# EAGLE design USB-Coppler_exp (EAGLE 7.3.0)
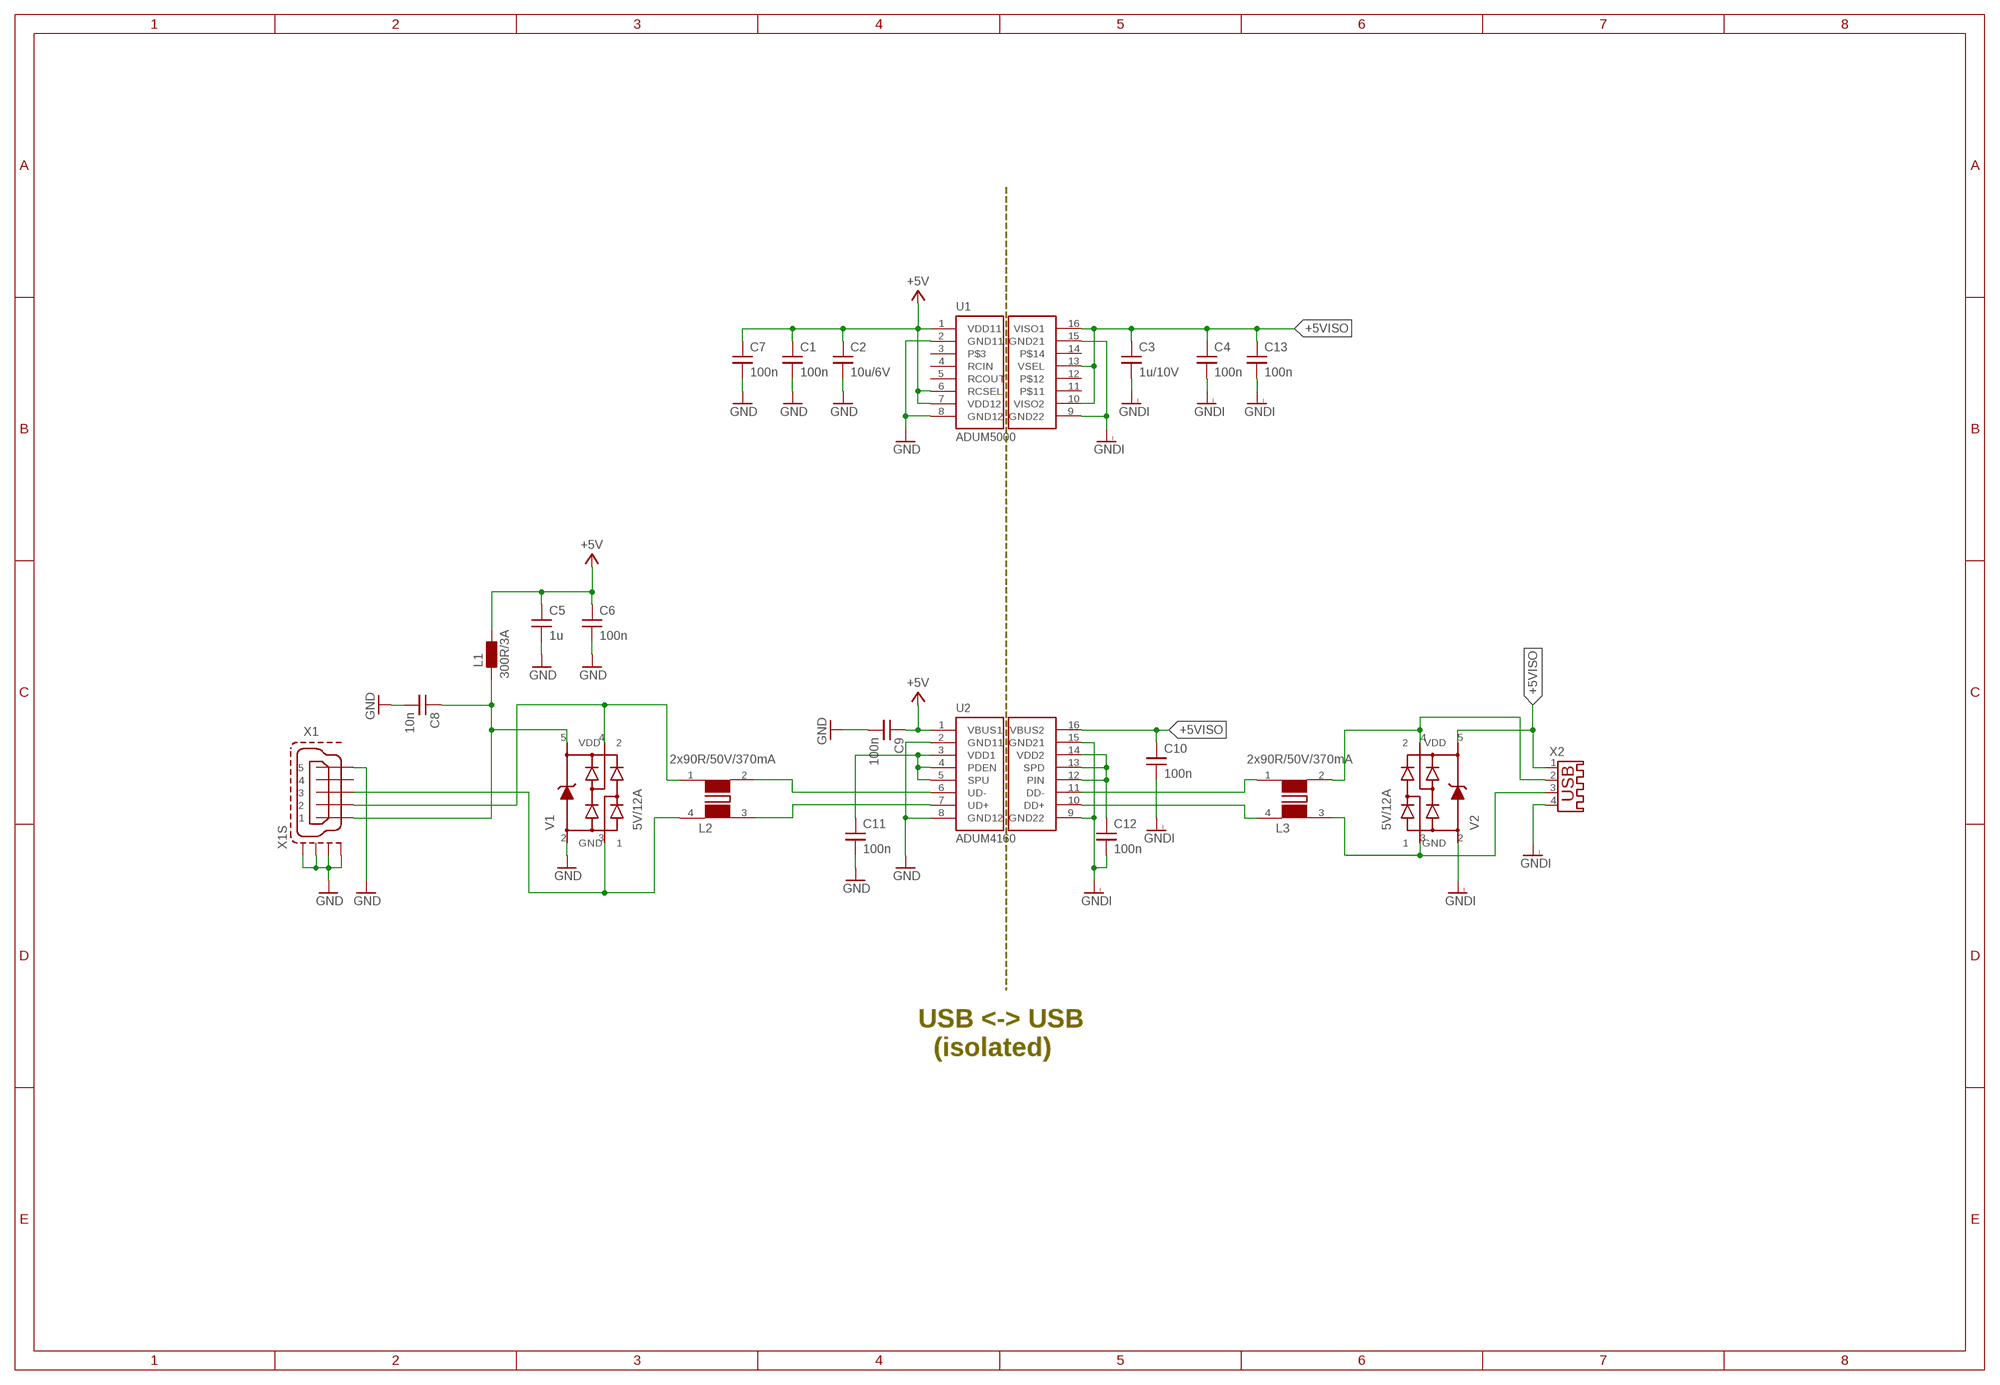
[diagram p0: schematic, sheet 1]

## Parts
C1  100n  C-EUC0603K  [C0603K]
C2  10u/6V  C-EUC0603K  [C0603K]
C3  1u/10V  C-EUC0603K  [C0603K]
C4  100n  C-EUC0603K  [C0603K]
C5  1u  C-EUC0603K  [C0603K]
C6  100n  C-EUC0603K  [C0603K]
C7  100n  C-EUC0603K  [C0603K]
C8  10n  C-EUC0603K  [C0603K]
C9  100n  C-EUC0603K  [C0603K]
C10  100n  C-EUC0603K  [C0603K]
C11  100n  C-EUC0603K  [C0603K]
C12  100n  C-EUC0603K  [C0603K]
C13  100n  C-EUC0603K  [C0603K]
L1  300R/3A  FERRIT-300R_3A  [0805]
L2  2x90R/50V/370mA  FILTER-C-WE-CNSW-1206_90R  [WE-CNSW_1206]
L3  2x90R/50V/370mA  FILTER-C-WE-CNSW-1206_90R  [WE-CNSW_1206]
U1  ADUM5000  [SOIC-16]
U2  ADUM4160  [SOIC-16]
V1  5V/12A  TVS_DIODE_WE-TVS_824011  [SOT23-5]
V2  5V/12A  TVS_DIODE_WE-TVS_824011  [SOT23-5]
X1  XB_MINIUSB_2486-01  [LUMBERG_2486_01]
X2  USB-A003  [USB-A003]

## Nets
+5V: C1.1 C2.1 C5.1 C6.1 C7.1 C9.1 L1.2 U1.1(VDD11) U1.6(RCSEL) U1.7(VDD12) U2.1(VBUS1)
+5VISO: C3.1 C4.1 C10.1 C13.1 U1.10(VISO2) U1.13(VSEL) U1.16(VISO1) U2.16(VBUS2) V2.5(VDD) X2.1
GND: C1.2 C2.2 C5.2 C6.2 C7.2 C8.2 C9.2 C11.2 U1.2(GND11) U1.8(GND12) U2.2(GND11) U2.8(GND12) V1.2(GND) X1.5 X1.M1(S1) X1.M2(S2) X1.M3(S3) X1.M4(S4)
GNDI: C3.2 C4.2 C10.2 C12.2 C13.2 U1.9(GND22) U1.15(GND21) U2.9(GND22) U2.15(GND21) V2.2(GND) X2.4
N$1: C11.1 U2.3(VDD1) U2.4(PDEN) U2.5(SPU)
N$2: L2.2 U2.6(UD-)
N$3: L2.3 U2.7(UD+)
N$5: C12.1 U2.12(PIN) U2.13(SPD) U2.14(VDD2)
N$6: L3.1 U2.11(DD-)
N$7: L3.4 U2.10(DD+)
N$8: L3.3 V2.3 X2.3
N$9: L3.2 V2.4 X2.2
N$531: L2.1 V1.4 X1.2
N$532: L2.4 V1.3 X1.3
N$533: C8.1 L1.1 V1.5(VDD) X1.1
Unconnected: U1.3 U1.4(RCIN) U1.5(RCOUT) U1.11 U1.12 U1.14 X1.4

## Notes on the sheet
- USB <-> USB
    (isolated)

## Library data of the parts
C1-C13 = LV_LG:C-EU: CAPACITOR, European symbol
L1 = 003-Schutzelemente:FERRIT; ARTIKELNR: 50107688; BEZEICHNUNG: Ferrit-C 300R@100MHz 3A 50mR; BEZEICHNUNG2: 742792031; HERSTELLER: WÜRTH
L2 L3 = 008-Filter:FILTER-C: SMD Common Mode Noise Suppressor WE_CNSW - Common mode data line filter - Wire wound -- USB 2.0 -- IEEE 1394 -- Power supply systems -- Signal interfaces; BEZEICHNUNG: Filter-C Datenleitungs-Filter (USB); BEZEICHNUNG2: 744232090; HERSTELLER: Würth
U1 = LV_LG:ADUM5000: FEATURES isoPower integrated, isolated dc-to-dc converter Regulated 3.3 V or 5 V output Up to 500 mW output power 16-lead SOIC package with 7.6 mm creepage High temperature operation: 105°C maximum Thermal overload protection
U2 = LV_LG:ADUM4160: FEATURES USB 2.0 compatible Low and full speed data rate: 1.5 Mbps and 12 Mbps Bidirectional communication 4.5 V to 5.5 V VBUSoperation 7 mA maximum upstream supply current @ 1.5 Mbps 8 mA maximum upstream supply current @ 12 Mbps 2.3 mA maximum upstream idle current Upstream short-circuit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
V1 V2 = 004-Dioden:TVS_DIODE_WE-TVS; ARTIKELNR: 50113145; BEZEICHNUNG: Diode-C WE-TVS Array; BEZEICHNUNG2: 824011 ESD-Protection; HERSTELLER: WUERTH
X1 = 009-Stecker:XB_MINIUSB_2486-01: MINI USB Connector Source: http://www.hirose.co.jp/cataloge_hp/e24000019.pdf; ARTIKELNR: n.v.; BEZEICHNUNG: Buchse Mini USB-B; BEZEICHNUNG2: 2486-01 (Bürklin 72F2280); HERSTELLER: Lumberg
X2 = con-yamaichi:USB-A003: USB connector; OC_FARNELL: unknown; OC_NEWARK: unknown

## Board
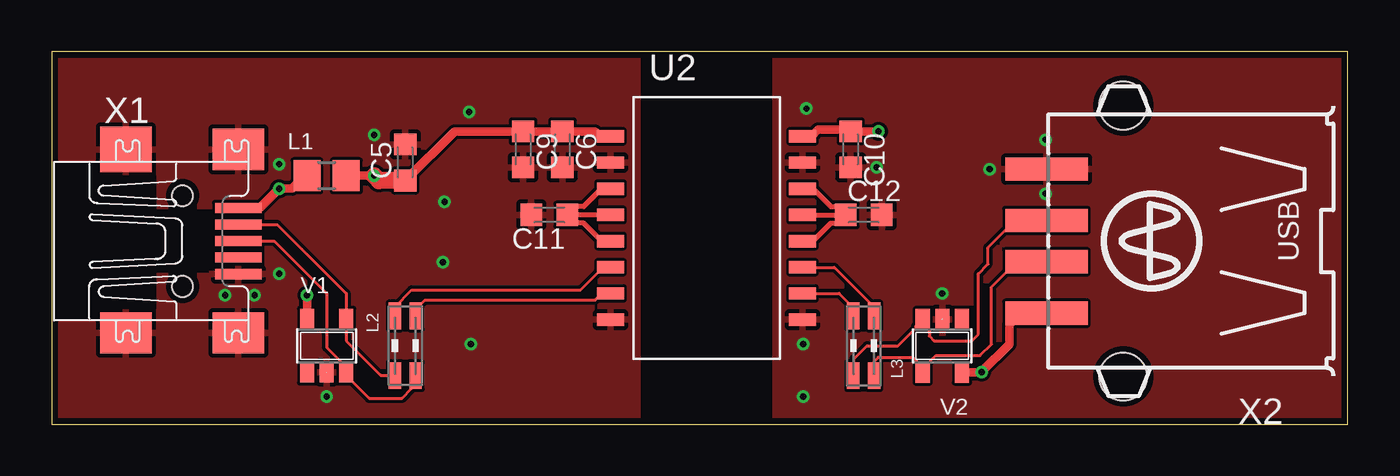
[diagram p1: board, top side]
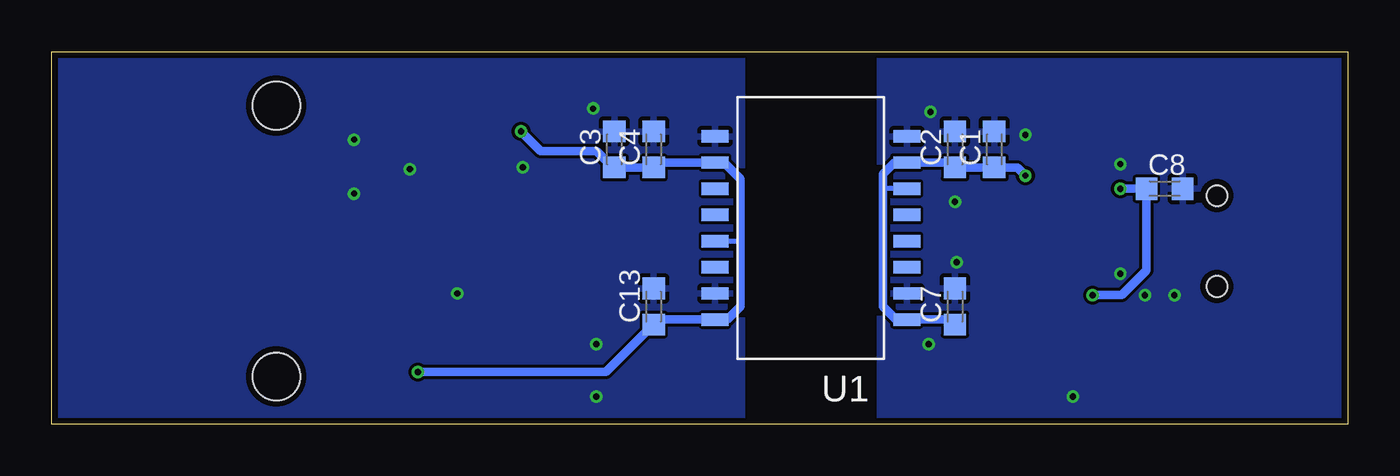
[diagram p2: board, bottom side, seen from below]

Size 62.84 x 18.09 mm. Coordinates in mm from the lower left corner, seen from the top.
Outline: 0,0 62.84,0 62.84,18.09 0,18.09 0,0
Copper layers (1*16): Top 0.035mm / dielectric 1.5mm / Bottom 0.035mm
Design rules "PCB-POOL Standard": minimum track width 0.15mm, minimum drill 0.3mm, track to track 0.15mm, track to pad 0.15mm, pad to pad 0.15mm, via to via 0.15mm, smd to smd 0.15mm, copper to edge 0.3mm, drill to drill 0.2mm, minimum pad ring 0.2mm, minimum via ring 0.15mm, stop-mask expansion 0.075mm, vias tented up to drill 0mil, thermal gap 0.2mm
tRestrict: area 28.6,0 to 34.9,18.4
bRestrict: area 22.9,0 to 29.2,18.4

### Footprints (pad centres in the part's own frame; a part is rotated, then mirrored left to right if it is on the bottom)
C0603K = smd 1.05 x 1.08: 1 -0.875,0; 2 0.875,0
0805 = smd 1.3 x 1.5: 1 -0.95,0; 2 0.95,0
WE-CNSW_1206 = smd 0.6 x 1.3: 1 -0.5,-1.45; 2 -0.5,1.45; 3 0.5,1.45; 4 0.5,-1.45
SOIC-16 = smd 0.6 x 1.3: 1 -4.445,-4.65; 2 -3.175,-4.65; 3 -1.905,-4.65; 4 -0.635,-4.65; 5 0.635,-4.65; 6 1.905,-4.65; 7 3.175,-4.65; 8 4.445,-4.65; 9 4.445,4.65; 10 3.175,4.65; 11 1.905,4.65; 12 0.635,4.65; 13 -0.635,4.65; 14 -1.905,4.65; 15 -3.175,4.65; 16 -4.445,4.65
SOT23-5 = smd 0.69 x 0.99: 1 -0.95,-1.29; 2 0,-1.29; 3 0.95,-1.29; 4 0.95,1.3; 5 -0.95,1.3
LUMBERG_2486_01 = smd 2.25 x 0.5: 1 2.7,1.6; 2 2.7,0.8; 3 2.7,0; 4 2.7,-0.8; 5 2.7,-1.6 | smd 2.5 x 2: M1 -2.75,-4.45; M3 2.7,4.45; M4 2.7,-4.45 | smd 2.5 x 2.2: M2 -2.75,4.45 | hole 1: 0,-2.2; 0,2.2
USB-A003 = smd 1.12 x 4: 1 -3.5,14; 2 -1,14; 3 1,14; 4 3.5,14 | hole 2.3: -6.57,10.28; 6.57,10.28

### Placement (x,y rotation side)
C1  17.14,13.34 90 bottom
C2  19.05,13.34 90 bottom
C3  35.56,13.34 90 bottom
C4  33.66,13.34 90 bottom
C5  17.14,12.7 90 top
C6  24.77,13.34 270 top
C7  19.05,5.71 90 bottom
C8  8.89,11.43 0 bottom
C9  22.86,13.34 270 top
C10  38.73,13.34 270 top
C11  24.13,10.16 180 top
C12  39.37,10.16 0 top
C13  33.66,5.71 90 bottom
L1  13.34,12.06 0 top
L2  17.14,3.81 0 top
L3  39.37,3.81 180 top
U1  26.04,9.53 90 bottom
U2  31.75,9.53 270 top
V1  13.34,3.81 0 top
V2  43.18,3.81 180 top
X1  6.35,8.89 0 top
X2  62.23,8.89 90 top

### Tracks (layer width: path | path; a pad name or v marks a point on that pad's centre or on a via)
+5V  (via drill 0.3)
  Top 0.406: L1.2 v15.64,12.06 | U2.1 26.59,13.97 26.35,14.21 C6.1 C9.1 19.53,14.21 C5.1
  Top 0.813: C5.1 15.88,11.82 v15.64,12.06
  Bottom 0.254: U1.6 22.54,11.43
  Bottom 0.406: v15.64,12.06 16.03,12.46 C1.1 C2.1 19.29,12.7 U1.7 21.99,12.7 22.54,12.14 22.54,11.43 22.54,5.71 21.91,5.08 U1.1 19.29,5.08 C7.1
+5VISO  (via drill 0.3)
  Top 0.406: v40.08,14.21 C10.1 38.66,14.29 37.15,14.29 36.83,13.97 U2.16 | V2.5 45.05,2.51 v45.09,2.54 46.43,3.89 46.43,4.84 46.98,5.39 X2.1
  Bottom 0.254: U1.13 29.45,8.89
  Bottom 0.406: v40.08,14.21 39.13,13.26 36.43,13.26 35.64,12.46 C3.1 C4.1 33.41,12.7 U1.10 30.24,12.7 29.45,11.91 29.45,8.89 29.45,5.71 30.08,5.08 U1.16 33.41,5.08 C13.1 35.96,2.54 v45.09,2.54
GND  (via drill 0.3)
  other vias: 15.64,14.05 11.03,12.62 11.03,7.3 9.84,6.27 8.41,6.27 18.97,7.86 20.32,3.89 20.24,15.16 19.05,10.79 13.34,1.35
  pour Top: 0,0 0,18.41 29.21,18.41 29.21,0
  pour Bottom: 0,0 0,18.41 23.5,18.41 23.5,0
GNDI  (via drill 0.3)
  other vias: 43.18,6.35 45.48,12.38 48.18,13.81 48.18,11.19 36.59,15.32 40.01,12.46 36.43,3.89 36.43,1.35
  pour Bottom: 28.57,0 28.57,18.41 62.87,18.41 62.87,0
  pour Top: 34.29,0 34.29,18.41 62.87,18.41 62.87,0
N$1
  Top 0.254: U2.5 26.67,8.89 25.8,9.76 25.4,9.76 C11.1 | U2.4 C11.1 | U2.3 26.67,11.43 25.8,10.56 25.32,10.56 C11.1
N$2
  Top 0.15: L2.2 16.64,5.69 17.46,6.51 25.64,6.51 26.51,7.38 26.51,7.46 26.59,7.54 27.02,7.54 U2.6
N$3
  Top 0.15: L2.3 17.64,5.58 18.1,6.03 26.35,6.03 26.59,6.27 27.02,6.27 U2.7
N$5
  Top 0.254: U2.14 36.91,11.43 37.78,10.56 38.1,10.56 C12.1 | U2.13 C12.1 | U2.12 36.91,8.89 37.78,9.76 38.1,9.77 C12.1
N$6
  Top 0.15: U2.11 37.94,7.62 39.77,5.79 39.77,5.36 L3.1
N$7
  Top 0.15: U2.10 38.18,6.35 38.73,5.79 38.73,5.39 L3.4
N$8
  Top 0.15: L3.3 38.87,2.75 38.89,2.86 38.89,3.17 39.53,3.81 41.04,3.81 41.91,4.68 41.91,4.78 V2.3 42.23,4.84 42.55,4.52 42.55,4.29 42.78,4.05 44.61,4.05 44.93,4.37 44.93,7.3 45.4,7.78 45.4,8.57 46.51,9.68 48.02,9.68 X2.3
N$9
  Top 0.15: X2.2 48.2,7.86 46.75,7.86 45.56,6.67 45.56,3.89 45.01,3.33 42.86,3.33 42.23,2.7 V2.4 41.99,2.75 41.99,3.02 41.75,3.25 40.08,3.25 39.87,3.04 L3.2
N$531
  Top 0.15: X1.2 10.95,9.69 14.29,6.35 V1.4 14.29,4.05 15.95,2.38 16.62,2.38 L2.1
N$532
  Top 0.15: X1.3 10.79,8.89 13.34,6.35 13.34,3.73 14.29,2.78 V1.3 | V1.3 | V1.3 14.29,2.38 15.4,1.27 16.99,1.27 17.46,1.75 17.46,2.18 L2.4
N$533  (via drill 0.3)
  Top 0.406: X1.1 10.09,10.49 v11.03,11.43 11.67,11.43 12.3,12.06 L1.1 | V1.5 v12.38,6.27
  Bottom 0.406: v11.03,11.43 C8.1 9.76,7.46 10.96,6.27 v12.38,6.27

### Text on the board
tStop: USB <-> USB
